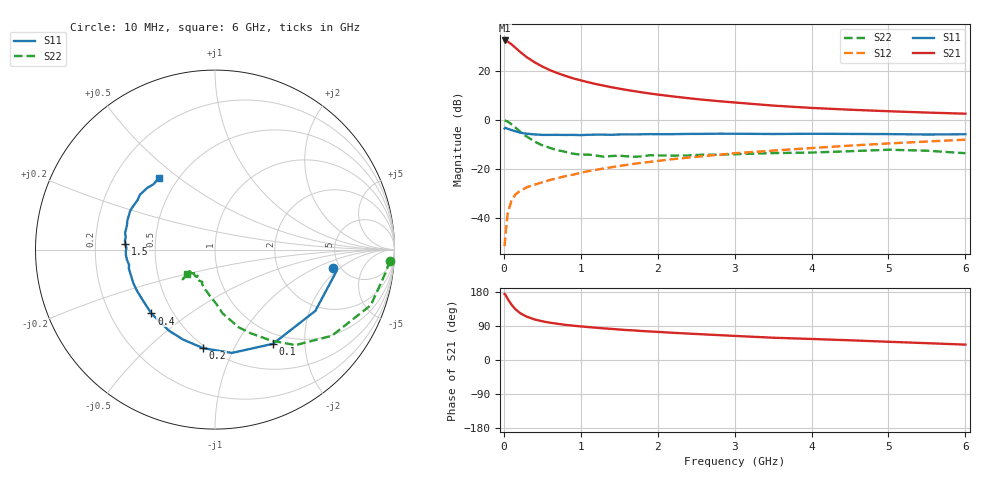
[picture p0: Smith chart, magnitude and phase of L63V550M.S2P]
!  INFINEON TECHNOLOGIES Small Signal Semiconductors
! BFR380L3 , Si-NPN RF-Transistor in TSLP-3-1
!  Vce=3.5 V,  Ic=50 mA
! Common Emitter S-Parameters:  07. March 2005
#  GHz  S  MA  R  50
! f  S11  S21  S12  S22
! GHz  Mag  Ang  Mag  Ang  Mag  Ang  Mag  Ang
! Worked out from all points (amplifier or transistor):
!   36 points, 10 MHz to 6 GHz, reference 50 ohm
!   highest |S21| = 32.5 dB at 10 MHz (marker M1)
!   |S21| within 3 dB of that: start of sweep to 151.5 MHz
!   unconditionally stable (mu >= 1): 1.584 GHz to 4.808 GHz
!   at 250 MHz: K = 0.47, MSG = 27.6 dB, |S12| = -28.5 dB
!   at 1.4 GHz: K = 0.99, MSG = 16.4 dB, |S12| = -19.4 dB
!   at 6 GHz: K = 0.97, MSG = 5.3 dB, |S12| = -8.1 dB
!   S11 on the Smith chart (normalised r, x): 10 MHz: 4.34, -1.60; 100 MHz: 0.85, -1.43; 200 MHz: 0.48, -0.76; 400 MHz: 0.38, -0.36; 1.5 GHz: 0.33, +0.03; 6 GHz: 0.39, +0.42
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0.01  0.6643 -8.9  42 174.3  0.0026 81.3  0.9759 -3.6
0.02  0.687 -10.2  41.88 172.5  0.0043 86.3  0.9583 -7.9
0.05  0.6551 -31.4  39.86 161.4  0.0122 77.4  0.9219 -19.6
0.1  0.6166 -58.3  34.97 146.0  0.0224 68.3  0.8091 -36.4
0.15  0.5834 -80.7  29.87 134.1  0.0296 59.0  0.6957 -49.9
0.2  0.5533 -96.8  25.41 125.5  0.0342 57.8  0.5948 -58.4
0.25  0.5317 -109.6  21.91 119.2  0.0377 54.3  0.5073 -66.8
0.3  0.5192 -119.8  19.01 114.2  0.0419 54.2  0.4529 -73.0
0.4  0.5024 -134.9  15.01 107.0  0.0471 54.3  0.358 -83.2
0.5  0.4915 -144.9  12.31 102.2  0.0527 55.8  0.3003 -88.9
0.6  0.4916 -152.4  10.36 98.4  0.0587 57.5  0.2659 -95.0
0.7  0.492 -157.6  8.997 95.5  0.0643 59.5  0.2386 -100.9
0.9  0.4914 -167.7  7.06 90.6  0.0754 61.5  0.2027 -110.8
1.1  0.4939 -173.4  5.847 86.8  0.0892 63.4  0.1945 -116.4
1.5  0.5012 176.5  4.34 80.4  0.1135 65.6  0.1843 -126.1
1.8  0.5061 170.6  3.64 76.4  0.1324 66.0  0.1788 -131.3
2.2  0.5091 164.5  3.005 71.8  0.157 66.1  0.1851 -134.0
2.8  0.5195 155.8  2.401 65.6  0.1933 65.9  0.1921 -140.2
3.5  0.5122 147.3  1.954 58.8  0.2346 63.9  0.2084 -138.8
4.5  0.5142 141.3  1.609 52.0  0.2965 62.2  0.2277 -138.1
5.5  0.5002 133.3  1.407 44.4  0.3594 58.4  0.2333 -137.6
6  0.5066 128.3  1.333 40.6  0.3919 56.2  0.2074 -139.5
